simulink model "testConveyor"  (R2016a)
settings: Solver=FixedStepDiscrete  StartTime=0.0  StopTime=20.1  RelTol=1e-3
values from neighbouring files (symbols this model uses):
  dt = block.DialogPrm(4).Data    [sfun_oven.m]
  t0 = block.DialogPrm(5).Data    [sfun_oven.m]
undefined symbols (not defined in the file or in its folder): m0, ndelay, newval, oldval
libraries: simulink x1

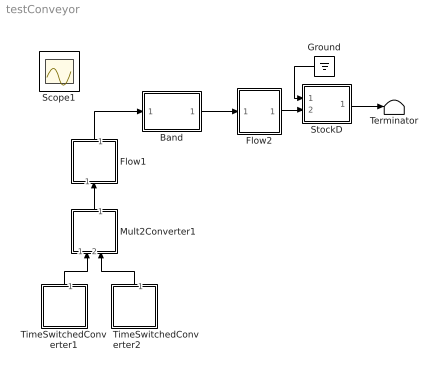
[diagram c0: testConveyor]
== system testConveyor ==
  Band : Subsystem
  Flow1 : Subsystem
  Flow2 : Subsystem
  Ground : Ground
  Mult2Converter1 : Subsystem
  StockD : Subsystem
  Terminator : Terminator
  TimeSwitchedConverter1 : Subsystem
  TimeSwitchedConverter2 : Subsystem
  Scope1 : Scope
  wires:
  Flow1/1(Out1) -> Band/1(In)
  Mult2Converter1/1(Out1) -> Flow1/1(In1)
  TimeSwitchedConverter1/1(Out1) -> Mult2Converter1/1(In1)
  TimeSwitchedConverter2/1(Out1) -> Mult2Converter1/2(In2)
  Band/1(Out) -> Flow2/1(In1)
  Flow2/1(Out1) -> StockD/2(In2)
  StockD/1(Out1) -> Terminator/1
  Ground/1 -> StockD/1(In1)

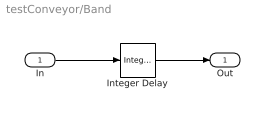
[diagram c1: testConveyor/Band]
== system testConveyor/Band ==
  In : Inport
  Integer Delay : simulink/Discrete/Integer Delay  NumDelays=ndelay  vinit=0.0  samptime=[dt,t0]
  Out : Outport
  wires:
  In/1 -> Integer Delay/1
  Integer Delay/1 -> Out/1

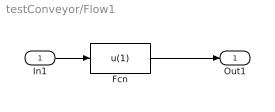
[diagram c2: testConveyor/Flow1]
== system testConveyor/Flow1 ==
  In1 : Inport
  Fcn : Fcn  Expr=u(1)
  Out1 : Outport
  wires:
  Fcn/1 -> Out1/1
  In1/1 -> Fcn/1

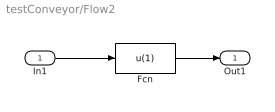
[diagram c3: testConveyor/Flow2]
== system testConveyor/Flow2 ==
  In1 : Inport
  Fcn : Fcn  Expr=u(1)
  Out1 : Outport
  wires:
  Fcn/1 -> Out1/1
  In1/1 -> Fcn/1

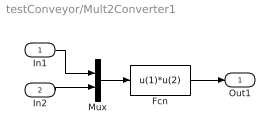
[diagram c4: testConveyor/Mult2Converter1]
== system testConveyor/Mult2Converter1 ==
  In1 : Inport
  In2 : Inport  Port=2
  Fcn : Fcn  Expr=u(1)*u(2)
  Mux : Mux  Inputs=2
  Out1 : Outport
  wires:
  Fcn/1 -> Out1/1
  Mux/1 -> Fcn/1
  In1/1 -> Mux/1
  In2/1 -> Mux/2

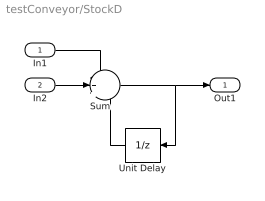
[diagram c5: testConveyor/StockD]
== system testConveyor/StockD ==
  In1 : Inport
  In2 : Inport  Port=2
  Sum : Sum  Inputs=-++
  Unit Delay : UnitDelay  InitialCondition=m0  SampleTime=[dt, t0]
  Out1 : Outport
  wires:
  In1/1 -> Sum/1
  Sum/1 -> Out1/1, Unit Delay/1
  In2/1 -> Sum/2
  Unit Delay/1 -> Sum/3

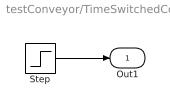
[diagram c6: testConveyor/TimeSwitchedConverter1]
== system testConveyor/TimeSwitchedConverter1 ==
  Step : Step  Time=t0  Before=oldval  After=newval
  Out1 : Outport
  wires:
  Step/1 -> Out1/1

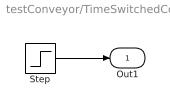
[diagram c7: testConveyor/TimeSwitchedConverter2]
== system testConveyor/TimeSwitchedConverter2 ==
  Step : Step  Time=t0  Before=oldval  After=newval
  Out1 : Outport
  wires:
  Step/1 -> Out1/1
